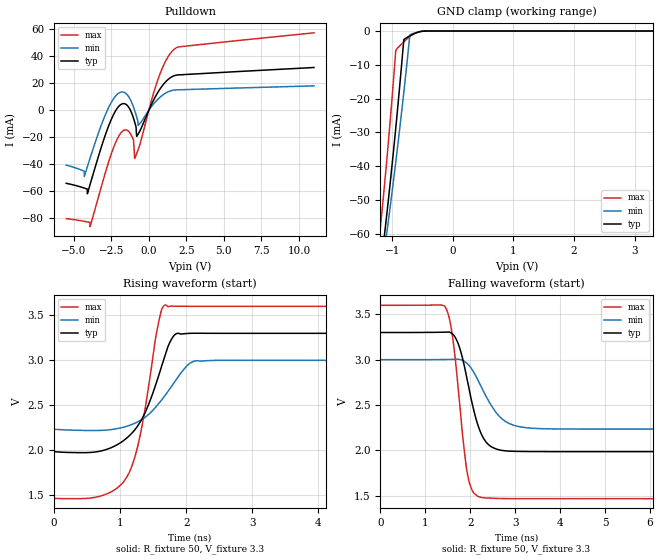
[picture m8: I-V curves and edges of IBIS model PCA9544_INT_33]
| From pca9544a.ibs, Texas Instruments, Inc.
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[Model]   PCA9544_INT_33
Model_type  Open_drain
Enable   Active-Low
Vref =   3.3V
Rref =   1k
Cref =   50p
Vmeas =   1.65
| variable   typ   min   max
C_comp   0.17pF   0.15pF   0.20pF
| C_pulldown   0.53pF   0.33pF   0.74pF
| C_tri-state   0.17pF   0.15pF   0.20pF
[Temperature Range]   40   100   -40
| Ambient temperature   25   85   -40
[Voltage range]   3.3   3   3.6
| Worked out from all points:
|   slope of the pulldown table from 0 to 0.495 V, typ, clamps not added: 44 ohm
|   GND clamp passes 1 mA (typ) near -0.66 V on its own axis
|   rising waveform, R_fixture 50, V_fixture 3.3: 20-80 % time 429ps typ, 495ps min, 312ps max; typ from 1.99 V to 3.3 V
|   falling waveform, R_fixture 50, V_fixture 3.3: 20-80 % time 374ps typ, 529ps min, 265ps max; typ from 3.3 V to 1.99 V
[GND Clamp]
| PCA9544_INT_33
|   Voltage   I(typ)   I(min)   I(max)
-5.5V     -353mA     -340.2mA   -363.4mA
-1.2V     -71.19mA   -74.19mA   -58.77mA
-1.125V   -59.7mA    -64.38mA   -44.86mA
-1.105V   -56.52mA   -61.69mA   -40.97mA
-1.09V    -54.11mA   -59.66mA   -37.99mA
-1.07V    -50.85mA   -56.93mA   -33.93mA
-945mV    -29.12mA   -39.11mA   -6.244mA
-940mV    -28.2mA    -38.37mA   -5.645mA
-810mV    -2.594mA   -18.16mA   -3.228mA
-710mV    -1.419mA   -1.185mA   -1.625mA
-485mV    -24.54uA   -33.77uA   -3.202uA
3.3V      17.67pA    41.36pA    13.24pA
[Pulldown]
| PCA9544_INT_33
|   Voltage   I(typ)   I(min)   I(max)
-5.5V     -54.16mA   -40.63mA   -80.34mA
-4.295V   -57.69mA   -49.06mA   -82.36mA
-3.91V    -55.05mA   -35.44mA   -86.27mA
-2.66V    -11.11mA   2.441mA    -37.76mA
-1.755V   4.855mA    13.6mA     -15.55mA
-1.02V    -5.812mA   2.457mA    -21.87mA
-935mV    -8.908mA   -298.4uA   -35.6mA
-810mV    -19.29mA   -4.806mA   -32.2mA
-705mV    -17.54mA   -11.23mA   -29.12mA
665mV     14.43mA    8.874mA    24.6mA
1.73V     25.81mA    15.11mA    45.63mA
11V       31.77mA    18.14mA    57.5mA
[Ramp]
| PCA9544_INT_33
| variable   typ   min   max
dV/dt_r   0.80/4.37E-10   0.47/5.15E-10   1.28/3.17E-10
dV/dt_f   0.79/3.78E-10   0.46/5.37E-10   1.28/2.68E-10
R_load = 50
[Rising Waveform]
| PCA9544_INT_33
R_fixture =   50
C_fixture =   0
L_fixture =   0
V_fixture =   3.3
V_fixture_min = 3
V_fixture_max = 3.6
|   Time   V(typ)   V(min)   V(max)
0s        1.986V     2.234V     1.467V
730ps     1.996V     2.222V     1.498V
1.115ns   2.145V     2.271V     1.719V
1.29ns    2.297V     2.325V     2.116V
1.565ns   2.784V     2.501V     3.353V
1.685ns   3.061V     2.614V     3.616V
1.855ns   3.297V     2.79V      3.602V
2.1ns     3.301V     2.985V     3.6V
2.475ns   3.3V       3V         3.6V
70ns      3.3V       3V         3.6V
[Falling Waveform]
| PCA9544_INT_33
R_fixture =   50
C_fixture =   0
L_fixture =   0
V_fixture =   3.3
V_fixture_min = 3
V_fixture_max = 3.6
|   Time   V(typ)   V(min)   V(max)
0s        3.3V       3V         3.6V
1.45ns    3.304V     3.002V     3.579V
1.62ns    3.279V     3.004V     3.211V
1.85ns    2.976V     2.987V     2.087V
1.96ns    2.718V     2.945V     1.69V
2.16ns    2.299V     2.789V     1.496V
2.355ns   2.091V     2.596V     1.474V
2.88ns    1.991V     2.294V     1.467V
3.91ns    1.986V     2.236V     1.467V
70ns      1.986V     2.234V     1.467V
